ORGANIZATION_BLOCK OB 1
TITLE = "Main Program Sweep (Cycle)"
VERSION : 0.1


VAR_TEMP
  OB1_EV_CLASS : BYTE ;	//Bits 0-3 = 1 (Coming event), Bits 4-7 = 1 (Event class 1)
  OB1_SCAN_1 : BYTE ;	//1 (Cold restart scan 1 of OB 1), 3 (Scan 2-n of OB 1)
  OB1_PRIORITY : BYTE ;	//Priority of OB Execution
  OB1_OB_NUMBR : BYTE ;	//1 (Organization block 1, OB1)
  OB1_RESERVED_1 : BYTE ;	//Reserved for system
  OB1_RESERVED_2 : BYTE ;	//Reserved for system
  OB1_PREV_CYCLE : INT ;	//Cycle time of previous OB1 scan (milliseconds)
  OB1_MIN_CYCLE : INT ;	//Minimum cycle time of OB1 (milliseconds)
  OB1_MAX_CYCLE : INT ;	//Maximum cycle time of OB1 (milliseconds)
  OB1_DATE_TIME : DATE_AND_TIME ;	//Date and time OB1 started
END_VAR
BEGIN
NETWORK
TITLE =Bit ON OFF
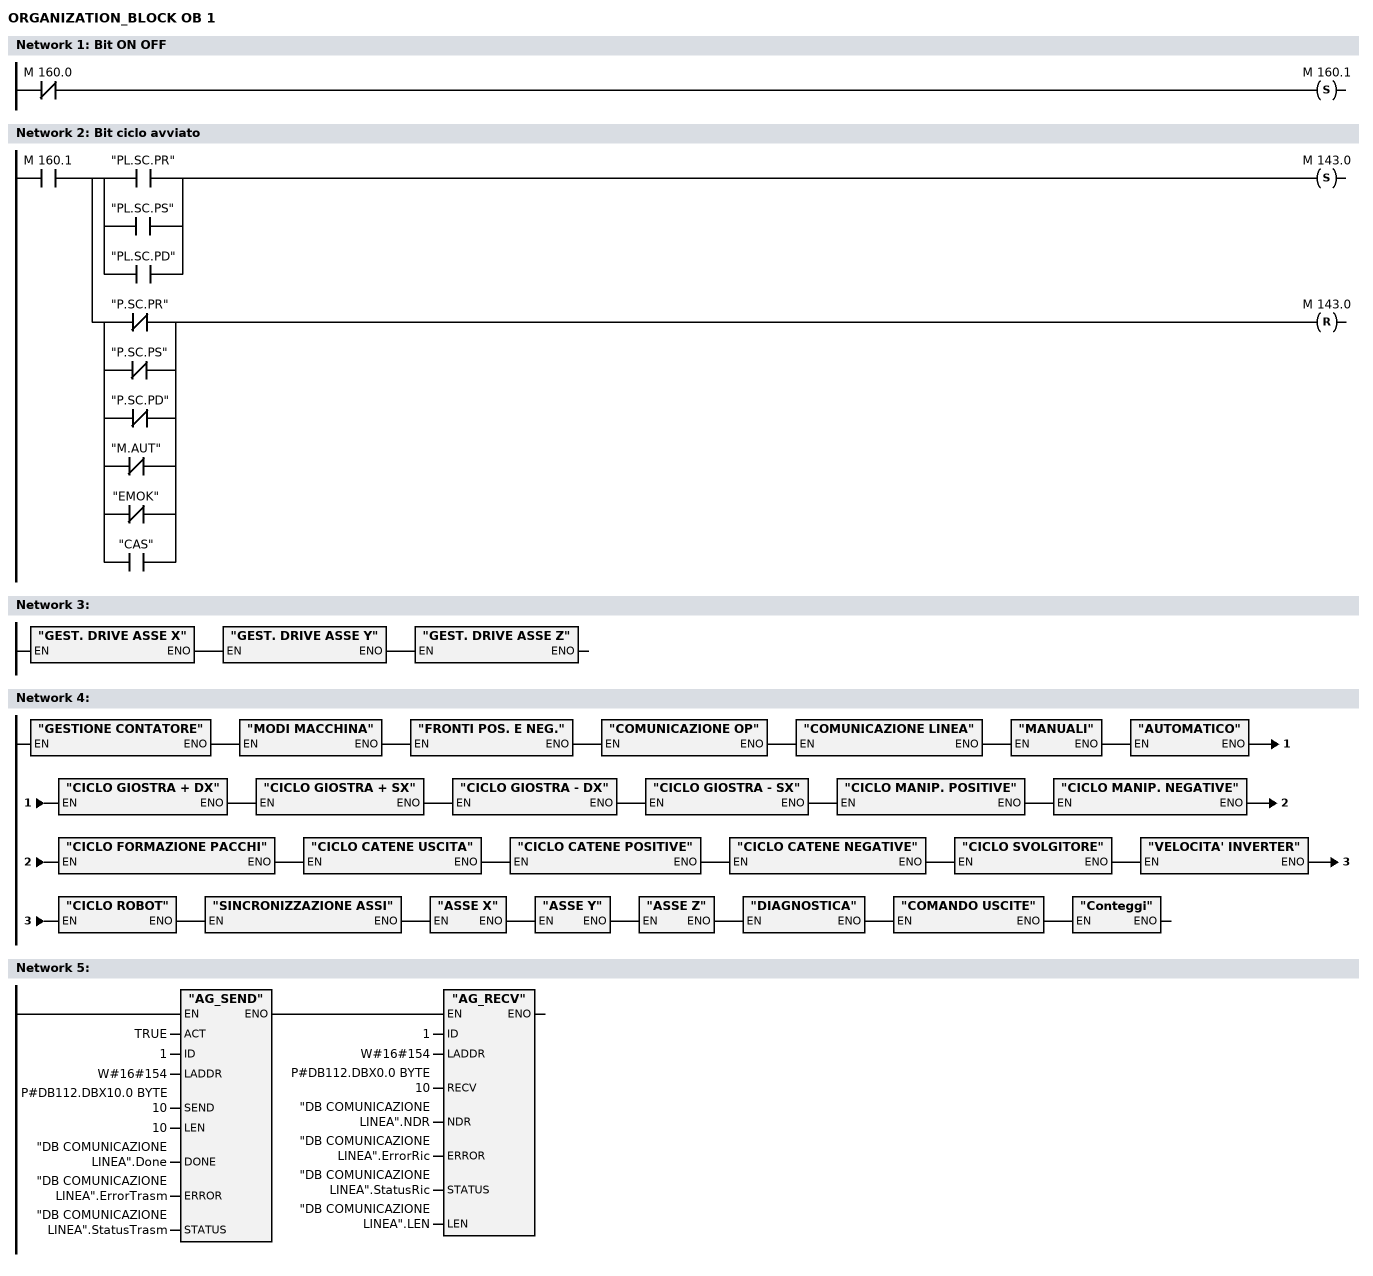
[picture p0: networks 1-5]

      UN    M    160.0;
      S     M    160.1;

NETWORK
TITLE =Bit ciclo avviato



      U     M    160.1;
      =     L     20.0;
      U     L     20.0;
      U(    ;
      O     "PL.SC.PR";
      O     "PL.SC.PS";
      O     "PL.SC.PD";
      )     ;
      S     M    143.0;
      U     L     20.0;
      U(    ;
      ON    "P.SC.PR";
      ON    "P.SC.PS";
      ON    "P.SC.PD";
      ON    "M.AUT";
      ON    "EMOK";
      O     "CAS";
      )     ;
      R     M    143.0;
NETWORK
TITLE =

      CALL "GEST. DRIVE ASSE X" ;
      CALL "GEST. DRIVE ASSE Y" ;
      CALL "GEST. DRIVE ASSE Z" ;


NETWORK
TITLE =

      CALL "GESTIONE CONTATORE" ;
      CALL "MODI MACCHINA" ;
      CALL "FRONTI POS. E NEG." ;
      CALL "COMUNICAZIONE OP" ;
      CALL "COMUNICAZIONE LINEA" ;
      CALL "MANUALI" ;
      CALL "AUTOMATICO" ;
      CALL "CICLO GIOSTRA + DX" ;
      CALL "CICLO GIOSTRA + SX" ;
      CALL "CICLO GIOSTRA - DX" ;
      CALL "CICLO GIOSTRA - SX" ;
      CALL "CICLO MANIP. POSITIVE" ;
      CALL "CICLO MANIP. NEGATIVE" ;
      CALL "CICLO FORMAZIONE PACCHI" ;
      CALL "CICLO CATENE USCITA" ;
      CALL "CICLO CATENE POSITIVE" ;
      CALL "CICLO CATENE NEGATIVE" ;
      CALL "CICLO SVOLGITORE" ;
      CALL "VELOCITA' INVERTER" ;
      CALL "CICLO ROBOT" ;
      CALL "SINCRONIZZAZIONE ASSI" ;
      CALL "ASSE X" ;
      CALL "ASSE Y" ;
      CALL "ASSE Z" ;
      CALL "DIAGNOSTICA" ;
      CALL "COMANDO USCITE" ;
      CALL "Conteggi" ;
NETWORK
TITLE =

      CALL "AG_SEND" (
           ACT                      := TRUE,
           ID                       := 1,
           LADDR                    := W#16#154,
           SEND                     := P#DB112.DBX10.0 BYTE 10,
           LEN                      := 10,
           DONE                     := "DB COMUNICAZIONE LINEA".Done,
           ERROR                    := "DB COMUNICAZIONE LINEA".ErrorTrasm,
           STATUS                   := "DB COMUNICAZIONE LINEA".StatusTrasm);
      CALL "AG_RECV" (
           ID                       := 1,
           LADDR                    := W#16#154,
           RECV                     := P#DB112.DBX0.0 BYTE 10,
           NDR                      := "DB COMUNICAZIONE LINEA".NDR,
           ERROR                    := "DB COMUNICAZIONE LINEA".ErrorRic,
           STATUS                   := "DB COMUNICAZIONE LINEA".StatusRic,
           LEN                      := "DB COMUNICAZIONE LINEA".LEN);
NETWORK
TITLE =

      SPA   M002;
      AUF   "DB DATI";
      L     P#26.0;
      LAR1  ;
      L     "DB DATI".PACCHI_DEPOSITATI;
      L     16;
      *I    ;
      +AR1  ;
      L     DBW [AR1,P#0.0];
      L     1;
      ==I   ;
      =     "CR.BR180°";
      U     "P.R.PR";
      FP    "CR.RRPP";
      SPBN  M001;
      L     "DB DATI".PACCHI_DEPOSITATI;
      L     1;
      +I    ;
      T     "DB DATI".PACCHI_DEPOSITATI;
M001: NOP   0;
      U     "TRT";
      SPBN  M002;
      L     0;
      T     "DB DATI".PACCHI_DEPOSITATI;
M002: NOP   0;
NETWORK
TITLE =
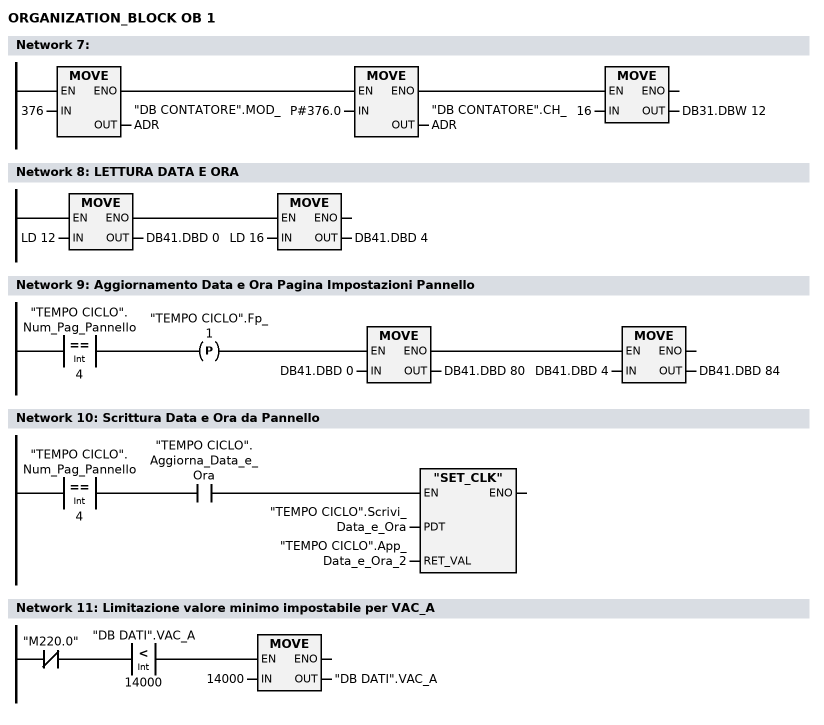
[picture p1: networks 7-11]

      L     376;
      T     "DB CONTATORE".MOD_ADR;
      L     P#376.0;
      T     "DB CONTATORE".CH_ADR;
      L     16;
      T     DB31.DBW   12;
NETWORK
TITLE =LETTURA DATA E ORA

      L     LD    12;
      T     DB41.DBD    0;

      L     LD    16;
      T     DB41.DBD    4;


NETWORK
TITLE =Aggiornamento Data e Ora Pagina Impostazioni Pannello

      L     "TEMPO CICLO".Num_Pag_Pannello;
      L     4;
      ==I   ;
      FP    "TEMPO CICLO".Fp_1;
      SPBN  s07;
      L     DB41.DBD    0;
      T     DB41.DBD   80;
      L     DB41.DBD    4;
      T     DB41.DBD   84;
s07:  NOP   0;

NETWORK
TITLE =Scrittura Data e Ora da Pannello

      L     "TEMPO CICLO".Num_Pag_Pannello;
      L     4;
      ==I   ;
      U     "TEMPO CICLO".Aggiorna_Data_e_Ora;
      SPBN  s08;
      CALL "SET_CLK" (
           PDT                      := "TEMPO CICLO".Scrivi_Data_e_Ora,
           RET_VAL                  := "TEMPO CICLO".App_Data_e_Ora_2);
      NOP   0;
s08:  NOP   0;
NETWORK
TITLE =Limitazione valore minimo impostabile per VAC_A




      UN    "M220.0";
      U(    ;
      L     "DB DATI".VAC_A;
      L     14000;
      <I    ;
      )     ;
      SPBNB _001;
      L     14000;
      T     "DB DATI".VAC_A;
_001: NOP   0;
END_ORGANIZATION_BLOCK

